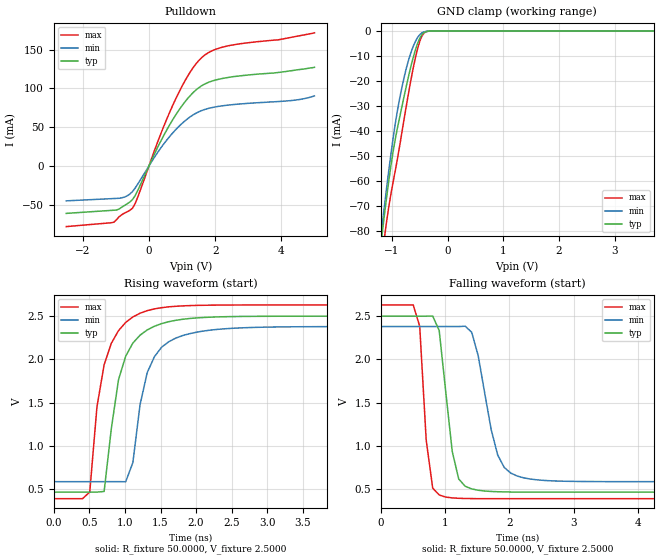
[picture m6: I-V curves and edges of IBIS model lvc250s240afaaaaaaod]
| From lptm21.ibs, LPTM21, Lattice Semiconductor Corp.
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|   Model lvc250s240afaaaaaaod
[Model]   lvc250s240afaaaaaaod
Model_type   I/O_open_drain
Polarity   Non-Inverting
Enable   Active-Low
Vinl =   0.7000V
Vinh =   1.7000V
Vmeas =   1.2500V
Cref =   0.0F
Rref =   1.0000M
Vref =   0.0V
C_comp   4.2000pF   3.8000pF   7.5000pF
[Temperature Range]   25.0000   0.1050k   -40.0000
[Voltage Range]   2.5000V   2.3800V   2.6300V
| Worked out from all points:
|   slope of the pulldown table from 0 to 0.375 V, typ, clamps not added: 11.2 ohm
|   GND clamp passes 1 mA (typ) near -0.44 V on its own axis
|   rising waveform, R_fixture 50.0000, V_fixture 2.5000: 20-80 % time 284ps typ, 277ps min, 263ps max; typ from 0.464 V to 2.5 V
|   falling waveform, R_fixture 50.0000, V_fixture 2.5000: 20-80 % time 188ps typ, 281ps min, 127ps max; typ from 2.5 V to 0.464 V
[Pulldown]
|Voltage   I(typ)   I(min)   I(max)
-2.5V     -61.25mA   -45.09mA   -78.29mA
-1.06V    -57.16mA   -42.08mA   -72.62mA
-740mV    -51.04mA   -40.26mA   -60.93mA
-500mV    -43.5mA    -33.15mA   -54.62mA
-340mV    -31.69mA   -23.47mA   -40.36mA
300mV     27.2mA     19.7mA     35.13mA
780mV     63.9mA     45.47mA    83.89mA
1.26V     91.34mA    63.75mA    122.1mA
1.66V     105.1mA    72.44mA    142.2mA
2.38V     114mA      78.38mA    154.8mA
4.3V      122.8mA    84.33mA    165.9mA
5V        127.2mA    90.33mA    171.7mA
[GND_clamp]
|Voltage   I(typ)   I(min)   I(max)
-2.5V     -564.7mA   -543.1mA   -585.2mA
-1.18V    -82.36mA   -79.04mA   -91.17mA
-1.14V    -74.89mA   -71.39mA   -83.98mA
-1.1V     -67.71mA   -63.95mA   -77.28mA
-980mV    -48.67mA   -43.37mA   -60.82mA
-820mV    -30.36mA   -22.66mA   -40.67mA
-700mV    -18.1mA    -11.63mA   -24.81mA
-620mV    -10.88mA   -6.341mA   -15.24mA
-540mV    -5.068mA   -2.657mA   -7.239mA
-460mV    -1.45mA    -716.2uA   -1.987mA
-300mV    -18.83uA   -15.98uA   -16.73uA
5V        0A         0A         0A
[Ramp]
| variable   typ   min   max
dV/dt_r  1.2215/0.2817n   1.0767/0.2741n   1.3449/0.2606n
dV/dt_f  1.2215/0.1862n   1.0767/0.2778n   1.3449/0.1259n
R_load = 50.0000
[Rising Waveform]
R_fixture=   50.0000
V_fixture=   2.5000
V_fixture_min=   2.3800
V_fixture_max=   2.6300
|time   V(typ)   V(min)   V(max)
0s        464.1mV    585.4mV    388.5mV
505.1ps   464.2mV    585.4mV    466.6mV
606.1ps   464.4mV    585.4mV    1.449V
707.1ps   472.4mV    585.4mV    1.938V
909.1ps   1.764V     585.8mV    2.332V
1.111ns   2.189V     806mV      2.491V
1.313ns   2.341V     1.847V     2.564V
1.616ns   2.436V     2.205V     2.608V
2.424ns   2.494V     2.355V     2.629V
10ns      2.5V       2.38V      2.63V
[Falling Waveform]
R_fixture=   50.0000
V_fixture=   2.5000
V_fixture_min=   2.3800
V_fixture_max=   2.6300
|time   V(typ)   V(min)   V(max)
0s        2.5V       2.38V      2.63V
505.1ps   2.5V       2.38V      2.63V
606.1ps   2.5V       2.38V      2.383V
808.1ps   2.502V     2.38V      510.7mV
1.01ns    1.629V     2.38V      407.1mV
1.212ns   616.4mV    2.38V      393.2mV
1.414ns   501.5mV    2.313V     389.7mV
1.818ns   469mV      893.2mV    388.6mV
2.222ns   464.9mV    629.6mV    388.6mV
10ns      464.2mV    585.4mV    388.5mV
